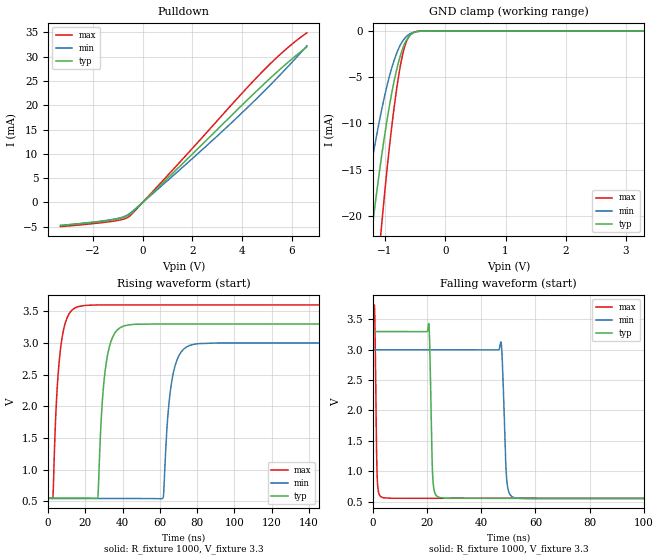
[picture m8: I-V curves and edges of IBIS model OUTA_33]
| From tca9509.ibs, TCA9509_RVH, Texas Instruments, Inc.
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[Model]   OUTA_33
Model_type  Open_drain
Enable   Active-High
Vref =   3.3
Rref =   1350
Cref =   50p
Vmeas =   1.65
| variable   typ   min   max
C_comp   2.27pF   1.68pF   2.57pF
| C_pulldown   1.51pF   1.17pF   1.73pF
| C_tri-state   2.27pF   1.68pF   2.57pF
[Temperature Range]   40   100   -40
| Ambient temperature   25   85   -40
[Voltage range]   3.3   3   3.6
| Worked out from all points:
|   slope of the pulldown table from 0 to 0.495 V, typ, clamps not added: 201 ohm
|   GND clamp passes 1 mA (typ) near -0.64 V on its own axis
|   rising waveform, R_fixture 1000, V_fixture 3.3: 20-80 % time 4.07ns typ, 4.42ns min, 3.78ns max; typ from 0.553 V to 3.3 V
|   falling waveform, R_fixture 1000, V_fixture 3.3: 20-80 % time 775ps typ, 1.11ns min, 536ps max; typ from 3.3 V to 0.553 V
[GND Clamp]
| OUTA_33
|   Voltage   I(typ)   I(min)   I(max)
-3.3V     -188.8mA   -139.3mA   -264.4mA
-1.405V   -32.52mA   -21.84mA   -49.76mA
-1.385V   -31.28mA   -20.97mA   -47.92mA
-1.22V    -21.72mA   -14.23mA   -33.54mA
-1.08V    -14.6mA    -9.277mA   -22.66mA
-1.055V   -13.44mA   -8.48mA    -20.86mA
-915mV    -7.645mA   -4.594mA   -11.82mA
-780mV    -3.455mA   -1.975mA   -5.083mA
-675mV    -1.388mA   -799.1uA   -1.701mA
-570mV    -376.8uA   -246.1uA   -331.7uA
-400mV    -16.68uA   -17.93uA   -5.645uA
3.3V      811.6pA    3.812nA    182.5pA
[Pulldown]
| OUTA_33
|   Voltage   I(typ)   I(min)   I(max)
-3.3V     -4.697mA   -4.747mA   -4.958mA
-1.245V   -3.611mA   -3.52mA    -3.894mA
-775mV    -3.1mA     -2.948mA   -3.44mA
-535mV    -2.544mA   -2.323mA   -2.863mA
880mV     4.37mA     3.953mA    4.861mA
2.5V      12.48mA    11.34mA    13.96mA
4.695V    23.48mA    21.94mA    26.29mA
5.695V    28.17mA    27.16mA    31.22mA
6.6V      32mA       32.21mA    34.89mA
[Ramp]
| OUTA_33
| variable   typ   min   max
dV/dt_r   1.65/4.07E-09   1.47/4.40E-09   1.83/3.78E-09
dV/dt_f   1.73/8.13E-10   1.55/1.18E-09   1.91/5.63E-10
R_load = 1000
[Rising Waveform]
| OUTA_33
R_fixture =   1000
C_fixture =   0
L_fixture =   0
V_fixture =   3.3
V_fixture_min = 3
V_fixture_max = 3.6
|   Time   V(typ)   V(min)   V(max)
0s        553.4mV    546.5mV    552.4mV
7.173ns   553.4mV    546.5mV    3.024V
15.94ns   553.4mV    546.5mV    3.572V
26.63ns   559.5mV    546.5mV    3.599V
31.17ns   2.683V     546.5mV    3.6V
40.32ns   3.265V     546.5mV    3.6V
61.76ns   3.3V       559.5mV    3.6V
66.57ns   3.3V       2.428V     3.6V
76.04ns   3.3V       2.961V     3.6V
267.2ns   3.3V       3V         3.6V
[Falling Waveform]
| OUTA_33
R_fixture =   1000
C_fixture =   0
L_fixture =   0
V_fixture =   3.3
V_fixture_min = 3
V_fixture_max = 3.6
|   Time   V(typ)   V(min)   V(max)
0s        3.3V       3V         3.6V
1.605ns   3.3V       3V         841.5mV
3.781ns   3.3V       3V         562.1mV
20.61ns   3.43V      3V         552.7mV
22.08ns   883.9mV    3V         552.7mV
24.64ns   566mV      3V         552.7mV
47.3ns    553.6mV    3.124V     552.7mV
49.42ns   553.6mV    843.8mV    552.7mV
52.43ns   553.6mV    561.2mV    552.7mV
267.2ns   553.4mV    546.6mV    552.5mV
